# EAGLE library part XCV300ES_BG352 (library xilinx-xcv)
xcv300es_bg352 edit this description Auto generated by make-symbol-device-package-bsdl.ulp Rev. 26 Source: xcv300es_bg352.bsd
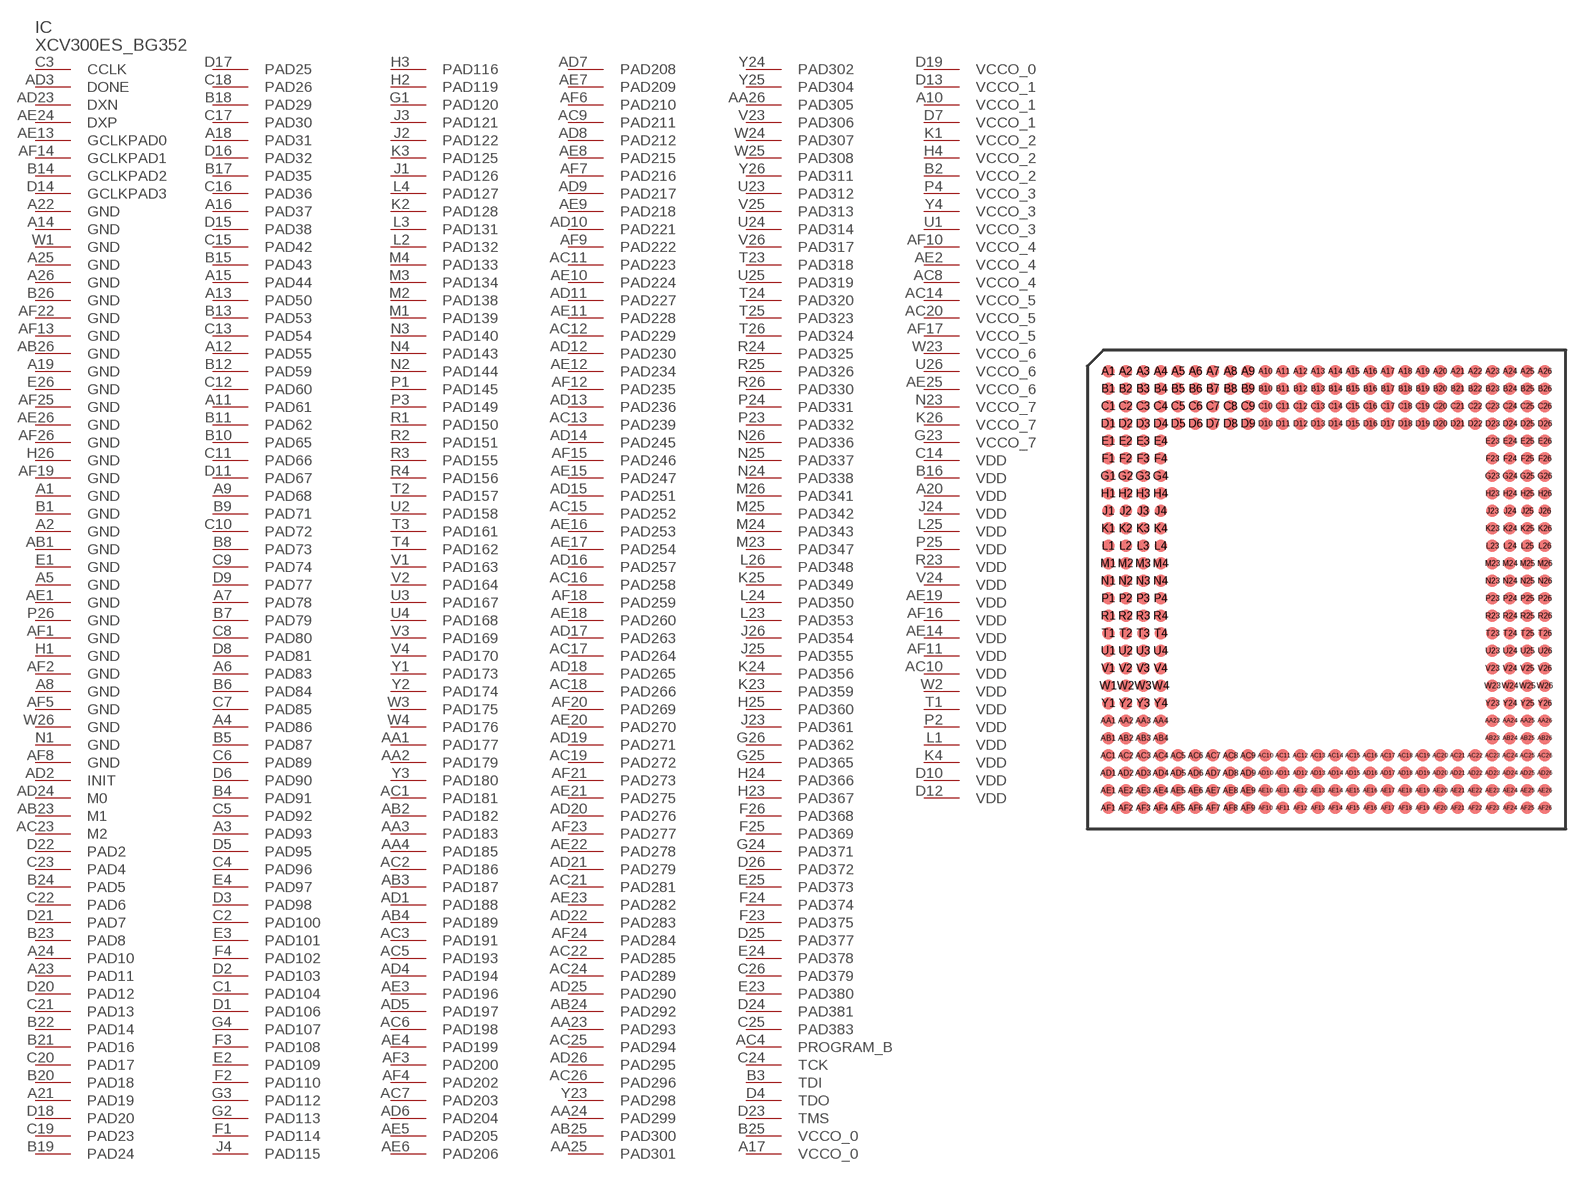
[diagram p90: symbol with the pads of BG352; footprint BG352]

Designator prefix IC

## XCV300ES_BG352 (OC_FARNELL: unknown; OC_NEWARK: unknown)  [BG352]
A1  GND  pwr
A2  GND  pwr
A3  PAD93
A4  PAD86
A5  GND  pwr
A6  PAD83
A7  PAD78
A8  GND  pwr
A9  PAD68
A10  VCCO_1  pwr
A11  PAD61
A12  PAD55
A13  PAD50
A14  GND  pwr
A15  PAD44
A16  PAD37
A17  VCCO_0  pwr
A18  PAD31
A19  GND  pwr
A20  VDD  pwr
A21  PAD19
A22  GND  pwr
A23  PAD11
A24  PAD10
A25  GND  pwr
A26  GND  pwr
AA1  PAD177
AA2  PAD179
AA3  PAD183
AA4  PAD185
AA23  PAD293
AA24  PAD299
AA25  PAD301
AA26  PAD305
AB1  GND  pwr
AB2  PAD182
AB3  PAD187
AB4  PAD189
AB23  M1  in
AB24  PAD292
AB25  PAD300
AB26  GND  pwr
AC1  PAD181
AC2  PAD186
AC3  PAD191
AC4  PROGRAM_B  in
AC5  PAD193
AC6  PAD198
AC7  PAD203
AC8  VCCO_4  pwr
AC9  PAD211
AC10  VDD  pwr
AC11  PAD223
AC12  PAD229
AC13  PAD239
AC14  VCCO_5  pwr
AC15  PAD252
AC16  PAD258
AC17  PAD264
AC18  PAD266
AC19  PAD272
AC20  VCCO_5  pwr
AC21  PAD281
AC22  PAD285
AC23  M2  in
AC24  PAD289
AC25  PAD294
AC26  PAD296
AD1  PAD188
AD2  INIT
AD3  DONE
AD4  PAD194
AD5  PAD197
AD6  PAD204
AD7  PAD208
AD8  PAD212
AD9  PAD217
AD10  PAD221
AD11  PAD227
AD12  PAD230
AD13  PAD236
AD14  PAD245
AD15  PAD251
AD16  PAD257
AD17  PAD263
AD18  PAD265
AD19  PAD271
AD20  PAD276
AD21  PAD279
AD22  PAD283
AD23  DXN  pas
AD24  M0  in
AD25  PAD290
AD26  PAD295
AE1  GND  pwr
AE2  VCCO_4  pwr
AE3  PAD196
AE4  PAD199
AE5  PAD205
AE6  PAD206
AE7  PAD209
AE8  PAD215
AE9  PAD218
AE10  PAD224
AE11  PAD228
AE12  PAD234
AE13  GCLKPAD0  in
AE14  VDD  pwr
AE15  PAD247
AE16  PAD253
AE17  PAD254
AE18  PAD260
AE19  VDD  pwr
AE20  PAD270
AE21  PAD275
AE22  PAD278
AE23  PAD282
AE24  DXP  pas
AE25  VCCO_6  pwr
AE26  GND  pwr
AF1  GND  pwr
AF2  GND  pwr
AF3  PAD200
AF4  PAD202
AF5  GND  pwr
AF6  PAD210
AF7  PAD216
AF8  GND  pwr
AF9  PAD222
AF10  VCCO_4  pwr
AF11  VDD  pwr
AF12  PAD235
AF13  GND  pwr
AF14  GCLKPAD1  in
AF15  PAD246
AF16  VDD  pwr
AF17  VCCO_5  pwr
AF18  PAD259
AF19  GND  pwr
AF20  PAD269
AF21  PAD273
AF22  GND  pwr
AF23  PAD277
AF24  PAD284
AF25  GND  pwr
AF26  GND  pwr
B1  GND  pwr
B2  VCCO_2  pwr
B3  TDI  in
B4  PAD91
B5  PAD87
B6  PAD84
B7  PAD79
B8  PAD73
B9  PAD71
B10  PAD65
B11  PAD62
B12  PAD59
B13  PAD53
B14  GCLKPAD2  in
B15  PAD43
B16  VDD  pwr
B17  PAD35
B18  PAD29
B19  PAD24
B20  PAD18
B21  PAD16
B22  PAD14
B23  PAD8
B24  PAD5
B25  VCCO_0  pwr
B26  GND  pwr
C1  PAD104
C2  PAD100
C3  CCLK
C4  PAD96
C5  PAD92
C6  PAD89
C7  PAD85
C8  PAD80
C9  PAD74
C10  PAD72
C11  PAD66
C12  PAD60
C13  PAD54
C14  VDD  pwr
C15  PAD42
C16  PAD36
C17  PAD30
C18  PAD26
C19  PAD23
C20  PAD17
C21  PAD13
C22  PAD6
C23  PAD4
C24  TCK  in
C25  PAD383
C26  PAD379
D1  PAD106
D2  PAD103
D3  PAD98
D4  TDO  out
D5  PAD95
D6  PAD90
D7  VCCO_1  pwr
D8  PAD81
D9  PAD77
D10  VDD  pwr
D11  PAD67
D12  VDD  pwr
D13  VCCO_1  pwr
D14  GCLKPAD3  in
D15  PAD38
D16  PAD32
D17  PAD25
D18  PAD20
D19  VCCO_0  pwr
D20  PAD12
D21  PAD7
D22  PAD2
D23  TMS  in
D24  PAD381
D25  PAD377
D26  PAD372
E1  GND  pwr
E2  PAD109
E3  PAD101
E4  PAD97
E23  PAD380
E24  PAD378
E25  PAD373
E26  GND  pwr
F1  PAD114
F2  PAD110
F3  PAD108
F4  PAD102
F23  PAD375
F24  PAD374
F25  PAD369
F26  PAD368
G1  PAD120
G2  PAD113
G3  PAD112
G4  PAD107
G23  VCCO_7  pwr
G24  PAD371
G25  PAD365
G26  PAD362
H1  GND  pwr
H2  PAD119
H3  PAD116
H4  VCCO_2  pwr
H23  PAD367
H24  PAD366
H25  PAD360
H26  GND  pwr
J1  PAD126
J2  PAD122
J3  PAD121
J4  PAD115
J23  PAD361
J24  VDD  pwr
J25  PAD355
J26  PAD354
K1  VCCO_2  pwr
K2  PAD128
K3  PAD125
K4  VDD  pwr
K23  PAD359
K24  PAD356
K25  PAD349
K26  VCCO_7  pwr
L1  VDD  pwr
L2  PAD132
L3  PAD131
L4  PAD127
L23  PAD353
L24  PAD350
L25  VDD  pwr
L26  PAD348
M1  PAD139
M2  PAD138
M3  PAD134
M4  PAD133
M23  PAD347
M24  PAD343
M25  PAD342
M26  PAD341
N1  GND  pwr
N2  PAD144
N3  PAD140
N4  PAD143
N23  VCCO_7  pwr
N24  PAD338
N25  PAD337
N26  PAD336
P1  PAD145
P2  VDD  pwr
P3  PAD149
P4  VCCO_3  pwr
P23  PAD332
P24  PAD331
P25  VDD  pwr
P26  GND  pwr
R1  PAD150
R2  PAD151
R3  PAD155
R4  PAD156
R23  VDD  pwr
R24  PAD325
R25  PAD326
R26  PAD330
T1  VDD  pwr
T2  PAD157
T3  PAD161
T4  PAD162
T23  PAD318
T24  PAD320
T25  PAD323
T26  PAD324
U1  VCCO_3  pwr
U2  PAD158
U3  PAD167
U4  PAD168
U23  PAD312
U24  PAD314
U25  PAD319
U26  VCCO_6  pwr
V1  PAD163
V2  PAD164
V3  PAD169
V4  PAD170
V23  PAD306
V24  VDD  pwr
V25  PAD313
V26  PAD317
W1  GND  pwr
W2  VDD  pwr
W3  PAD175
W4  PAD176
W23  VCCO_6  pwr
W24  PAD307
W25  PAD308
W26  GND  pwr
Y1  PAD173
Y2  PAD174
Y3  PAD180
Y4  VCCO_3  pwr
Y23  PAD298
Y24  PAD302
Y25  PAD304
Y26  PAD311

## Footprint BG352 (pad centres in mm)
xcv100e_bg352 edit this description Auto generated by make-symbol-device-package-bsdl.ulp Rev. 26 Source: xcv100e_bg352.bsd
smd 0.9 x 0.9: A1 -15.875,15.875; A2 -14.605,15.875; A3 -13.335,15.875; A4 -12.065,15.875; A5 -10.795,15.875; A6 -9.525,15.875; A7 -8.255,15.875; A8 -6.985,15.875; A9 -5.715,15.875; A10 -4.445,15.875; A11 -3.175,15.875; A12 -1.905,15.875; A13 -0.635,15.875; A14 0.635,15.875; A15 1.905,15.875; A16 3.175,15.875; A17 4.445,15.875; A18 5.715,15.875; A19 6.985,15.875; A20 8.255,15.875; A21 9.525,15.875; A22 10.795,15.875; A23 12.065,15.875; A24 13.335,15.875; A25 14.605,15.875; A26 15.875,15.875; AA1 -15.875,-9.525; AA2 -14.605,-9.525; AA3 -13.335,-9.525; AA4 -12.065,-9.525; AA23 12.065,-9.525; AA24 13.335,-9.525; AA25 14.605,-9.525; AA26 15.875,-9.525; AB1 -15.875,-10.795; AB2 -14.605,-10.795; AB3 -13.335,-10.795; AB4 -12.065,-10.795; AB23 12.065,-10.795; AB24 13.335,-10.795; AB25 14.605,-10.795; AB26 15.875,-10.795; AC1 -15.875,-12.065; AC2 -14.605,-12.065; AC3 -13.335,-12.065; AC4 -12.065,-12.065; AC5 -10.795,-12.065; AC6 -9.525,-12.065; AC7 -8.255,-12.065; AC8 -6.985,-12.065; AC9 -5.715,-12.065; AC10 -4.445,-12.065; AC11 -3.175,-12.065; AC12 -1.905,-12.065; AC13 -0.635,-12.065; AC14 0.635,-12.065; AC15 1.905,-12.065; AC16 3.175,-12.065; AC17 4.445,-12.065; AC18 5.715,-12.065; AC19 6.985,-12.065; AC20 8.255,-12.065; AC21 9.525,-12.065; AC22 10.795,-12.065; AC23 12.065,-12.065; AC24 13.335,-12.065; AC25 14.605,-12.065; AC26 15.875,-12.065; AD1 -15.875,-13.335; AD2 -14.605,-13.335; AD3 -13.335,-13.335; AD4 -12.065,-13.335; AD5 -10.795,-13.335; AD6 -9.525,-13.335; AD7 -8.255,-13.335; AD8 -6.985,-13.335; AD9 -5.715,-13.335; AD10 -4.445,-13.335; AD11 -3.175,-13.335; AD12 -1.905,-13.335; AD13 -0.635,-13.335; AD14 0.635,-13.335; AD15 1.905,-13.335; AD16 3.175,-13.335; AD17 4.445,-13.335; AD18 5.715,-13.335; AD19 6.985,-13.335; AD20 8.255,-13.335; AD21 9.525,-13.335; AD22 10.795,-13.335; AD23 12.065,-13.335; AD24 13.335,-13.335; AD25 14.605,-13.335; AD26 15.875,-13.335; AE1 -15.875,-14.605; AE2 -14.605,-14.605; AE3 -13.335,-14.605; AE4 -12.065,-14.605; AE5 -10.795,-14.605; AE6 -9.525,-14.605; AE7 -8.255,-14.605; AE8 -6.985,-14.605; AE9 -5.715,-14.605; AE10 -4.445,-14.605; AE11 -3.175,-14.605; AE12 -1.905,-14.605; AE13 -0.635,-14.605; AE14 0.635,-14.605; AE15 1.905,-14.605; AE16 3.175,-14.605; AE17 4.445,-14.605; AE18 5.715,-14.605; AE19 6.985,-14.605; AE20 8.255,-14.605; AE21 9.525,-14.605; AE22 10.795,-14.605; AE23 12.065,-14.605; AE24 13.335,-14.605; AE25 14.605,-14.605; AE26 15.875,-14.605; AF1 -15.875,-15.875; AF2 -14.605,-15.875; AF3 -13.335,-15.875; AF4 -12.065,-15.875; AF5 -10.795,-15.875; AF6 -9.525,-15.875; AF7 -8.255,-15.875; AF8 -6.985,-15.875; AF9 -5.715,-15.875; AF10 -4.445,-15.875; AF11 -3.175,-15.875; AF12 -1.905,-15.875; AF13 -0.635,-15.875; AF14 0.635,-15.875; AF15 1.905,-15.875; AF16 3.175,-15.875; AF17 4.445,-15.875; AF18 5.715,-15.875; AF19 6.985,-15.875; AF20 8.255,-15.875; AF21 9.525,-15.875; AF22 10.795,-15.875; AF23 12.065,-15.875; AF24 13.335,-15.875; AF25 14.605,-15.875; AF26 15.875,-15.875; B1 -15.875,14.605; B2 -14.605,14.605; B3 -13.335,14.605; B4 -12.065,14.605; B5 -10.795,14.605; B6 -9.525,14.605; B7 -8.255,14.605; B8 -6.985,14.605; B9 -5.715,14.605; B10 -4.445,14.605; B11 -3.175,14.605; B12 -1.905,14.605; B13 -0.635,14.605; B14 0.635,14.605; B15 1.905,14.605; B16 3.175,14.605; B17 4.445,14.605; B18 5.715,14.605; B19 6.985,14.605; B20 8.255,14.605; B21 9.525,14.605; B22 10.795,14.605; B23 12.065,14.605; B24 13.335,14.605; B25 14.605,14.605; B26 15.875,14.605; C1 -15.875,13.335; C2 -14.605,13.335; C3 -13.335,13.335; C4 -12.065,13.335; C5 -10.795,13.335; C6 -9.525,13.335; C7 -8.255,13.335; C8 -6.985,13.335; C9 -5.715,13.335; C10 -4.445,13.335; C11 -3.175,13.335; C12 -1.905,13.335; C13 -0.635,13.335; C14 0.635,13.335; C15 1.905,13.335; C16 3.175,13.335; C17 4.445,13.335; C18 5.715,13.335; C19 6.985,13.335; C20 8.255,13.335; C21 9.525,13.335; C22 10.795,13.335; C23 12.065,13.335; C24 13.335,13.335; C25 14.605,13.335; C26 15.875,13.335; D1 -15.875,12.065; D2 -14.605,12.065; D3 -13.335,12.065; D4 -12.065,12.065; D5 -10.795,12.065; D6 -9.525,12.065; D7 -8.255,12.065; D8 -6.985,12.065; D9 -5.715,12.065; D10 -4.445,12.065; D11 -3.175,12.065; D12 -1.905,12.065; D13 -0.635,12.065; D14 0.635,12.065; D15 1.905,12.065; D16 3.175,12.065; D17 4.445,12.065; D18 5.715,12.065; D19 6.985,12.065; D20 8.255,12.065; D21 9.525,12.065; D22 10.795,12.065; D23 12.065,12.065; D24 13.335,12.065; D25 14.605,12.065; D26 15.875,12.065; E1 -15.875,10.795; E2 -14.605,10.795; E3 -13.335,10.795; E4 -12.065,10.795; E23 12.065,10.795; E24 13.335,10.795; E25 14.605,10.795; E26 15.875,10.795; F1 -15.875,9.525; F2 -14.605,9.525; F3 -13.335,9.525; F4 -12.065,9.525; F23 12.065,9.525; F24 13.335,9.525; F25 14.605,9.525; F26 15.875,9.525; G1 -15.875,8.255; G2 -14.605,8.255; G3 -13.335,8.255; G4 -12.065,8.255; G23 12.065,8.255; G24 13.335,8.255; G25 14.605,8.255; G26 15.875,8.255; H1 -15.875,6.985; H2 -14.605,6.985; H3 -13.335,6.985; H4 -12.065,6.985; H23 12.065,6.985; H24 13.335,6.985; H25 14.605,6.985; H26 15.875,6.985; J1 -15.875,5.715; J2 -14.605,5.715; J3 -13.335,5.715; J4 -12.065,5.715; J23 12.065,5.715; J24 13.335,5.715; J25 14.605,5.715; J26 15.875,5.715; K1 -15.875,4.445; K2 -14.605,4.445; K3 -13.335,4.445; K4 -12.065,4.445; K23 12.065,4.445; K24 13.335,4.445; K25 14.605,4.445; K26 15.875,4.445; L1 -15.875,3.175; L2 -14.605,3.175; L3 -13.335,3.175; L4 -12.065,3.175; L23 12.065,3.175; L24 13.335,3.175; L25 14.605,3.175; L26 15.875,3.175; M1 -15.875,1.905; M2 -14.605,1.905; M3 -13.335,1.905; M4 -12.065,1.905; M23 12.065,1.905; M24 13.335,1.905; M25 14.605,1.905; M26 15.875,1.905; N1 -15.875,0.635; N2 -14.605,0.635; N3 -13.335,0.635; N4 -12.065,0.635; N23 12.065,0.635; N24 13.335,0.635; N25 14.605,0.635; N26 15.875,0.635; P1 -15.875,-0.635; P2 -14.605,-0.635; P3 -13.335,-0.635; P4 -12.065,-0.635; P23 12.065,-0.635; P24 13.335,-0.635; P25 14.605,-0.635; P26 15.875,-0.635; R1 -15.875,-1.905; R2 -14.605,-1.905; R3 -13.335,-1.905; R4 -12.065,-1.905; R23 12.065,-1.905; R24 13.335,-1.905; R25 14.605,-1.905; R26 15.875,-1.905; T1 -15.875,-3.175; T2 -14.605,-3.175; T3 -13.335,-3.175; T4 -12.065,-3.175; T23 12.065,-3.175; T24 13.335,-3.175; T25 14.605,-3.175; T26 15.875,-3.175; U1 -15.875,-4.445; U2 -14.605,-4.445; U3 -13.335,-4.445; U4 -12.065,-4.445; U23 12.065,-4.445; U24 13.335,-4.445; U25 14.605,-4.445; U26 15.875,-4.445; V1 -15.875,-5.715; V2 -14.605,-5.715; V3 -13.335,-5.715; V4 -12.065,-5.715; V23 12.065,-5.715; V24 13.335,-5.715; V25 14.605,-5.715; V26 15.875,-5.715; W1 -15.875,-6.985; W2 -14.605,-6.985; W3 -13.335,-6.985; W4 -12.065,-6.985; W23 12.065,-6.985; W24 13.335,-6.985; W25 14.605,-6.985; W26 15.875,-6.985; Y1 -15.875,-8.255; Y2 -14.605,-8.255; Y3 -13.335,-8.255; Y4 -12.065,-8.255; Y23 12.065,-8.255; Y24 13.335,-8.255; Y25 14.605,-8.255; Y26 15.875,-8.255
